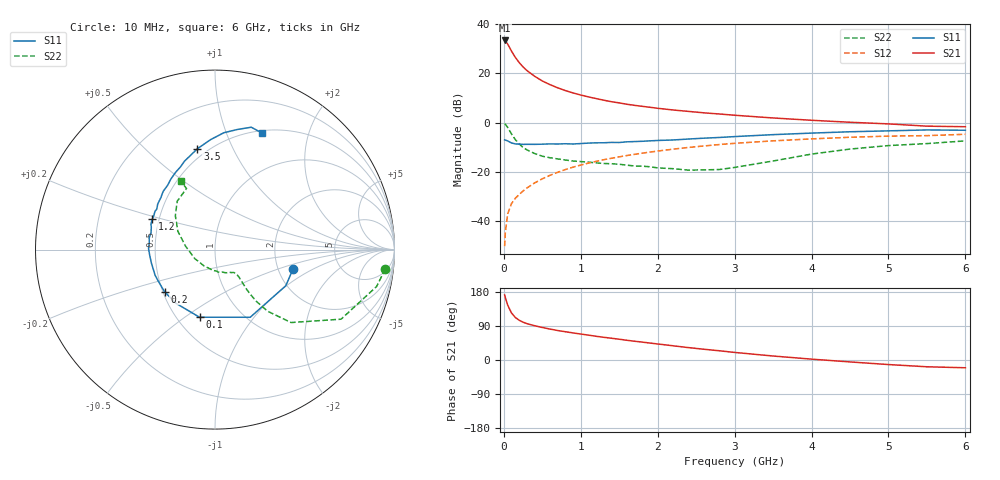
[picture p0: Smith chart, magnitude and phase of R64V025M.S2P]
! SIEMENS Small Signal Semiconductors
! BFR193
! Si NPN RF Bipolar Junction Transistor in SOT23
! VCE = 4 V  IC = 25 mA
! Common Emitter S-Parameters:  May  1996
# GHz  S  MA  R  50
!  f  S11  S21  S12  S22
! GHz  MAG  ANG  MAG  ANG  MAG  ANG  MAG  ANG
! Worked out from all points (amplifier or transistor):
!   36 points, 10 MHz to 6 GHz, reference 50 ohm
!   highest |S21| = 33.4 dB at 10 MHz (marker M1)
!   |S21| within 3 dB of that: start of sweep to 76.66 MHz
!   unconditionally stable (mu >= 1): 512.3 MHz to 1.907 GHz
!   at 250 MHz: K = 0.87, MSG = 25.2 dB, |S12| = -27.8 dB
!   at 1.4 GHz: K = 1.02, MAG = 10.5 dB, |S12| = -14.5 dB
!   at 6 GHz: K = 0.95, MSG = 1.5 dB, |S12| = -4.7 dB
!   S11 on the Smith chart (normalised r, x): 10 MHz: 2.40, -0.66; 100 MHz: 0.64, -0.57; 200 MHz: 0.51, -0.28; 1.2 GHz: 0.46, +0.19; 3.5 GHz: 0.44, +0.74; 6 GHz: 0.53, +1.34
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0.01  0.4476 -14.2  46.66 171.9  0.0031 85.6  0.9549 -6.5
0.02  0.443 -27.0  45.28 164.2  0.006 78.7  0.9232 -12.9
0.05  0.425 -62.5  39.38 144.7  0.014 71.2  0.8023 -28.9
0.1  0.3865 -102.9  28.32 124.0  0.0228 64.3  0.5871 -43.8
0.15  0.3698 -125.9  21.04 112.1  0.0292 64.1  0.4512 -49.5
0.2  0.3662 -140.2  16.57 104.9  0.0348 65.8  0.3682 -51.4
0.25  0.3616 -150.2  13.52 99.8  0.0409 66.8  0.3135 -51.7
0.3  0.3631 -156.7  11.42 96.0  0.0471 68.4  0.2802 -51.4
0.4  0.3622 -168.1  8.749 90.4  0.0596 70.0  0.236 -50.2
0.5  0.3652 -175.1  7.022 85.8  0.0724 70.4  0.2081 -49.1
0.6  0.3701 179.3  5.905 81.6  0.0851 70.7  0.1935 -48.7
0.7  0.3683 173.7  5.099 77.8  0.0981 70.1  0.1835 -49.2
0.8  0.3726 169.9  4.476 74.6  0.1114 69.4  0.1743 -49.7
0.9  0.3683 165.4  4.006 71.4  0.1248 68.6  0.1662 -50.3
1.1  0.3844 158.2  3.332 65.6  0.1508 67.0  0.1577 -54.4
1.2  0.389 153.6  3.08 62.6  0.1637 65.9  0.1522 -56.4
1.6  0.4078 141.5  2.362 52.0  0.2149 60.8  0.1367 -68.5
2.2  0.4447 126.5  1.808 37.5  0.2894 52.5  0.1161 -96.3
3.5  0.5705 99.9  1.244 10.5  0.4266 32.7  0.1663 172.9
4.5  0.6528 85.7  1.018 -5.1  0.5047 18.5  0.2906 139.5
5.5  0.7111 73.5  0.848 -17.9  0.5444 4.4  0.3754 115.0
6  0.7005 68.1  0.826 -20.5  0.5805 0.3  0.4262 116.6
